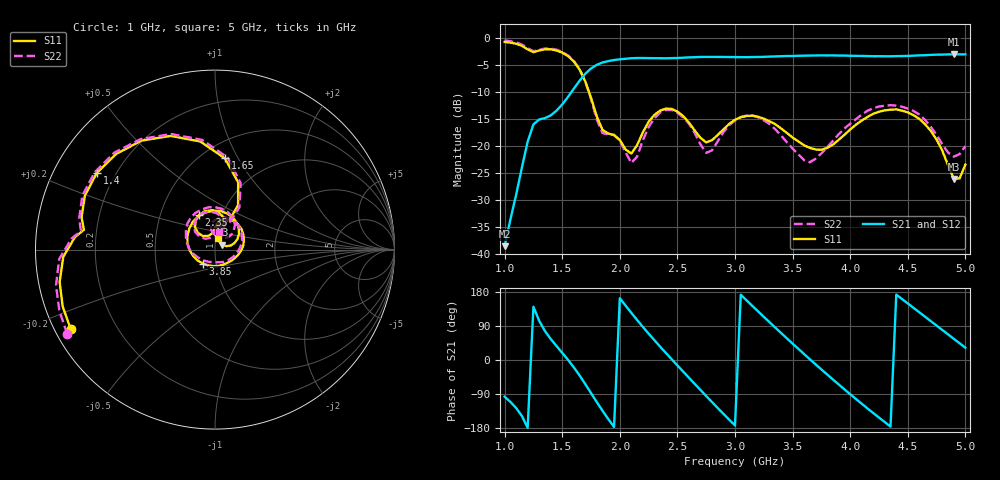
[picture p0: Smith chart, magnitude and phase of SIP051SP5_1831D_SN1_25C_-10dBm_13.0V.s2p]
# GHz  S  dB  R  50
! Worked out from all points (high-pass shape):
!   81 points, 1 GHz to 5 GHz, reference 50 ohm
!   highest |S21| = -3.03 dB at 4.9 GHz (marker M1); lowest = -38.6 dB at 1 GHz (marker M2)
!   |S21| within 3 dB of the highest: 1.731 GHz to end of sweep
!   lowest |S11| = -26.1 dB at 4.9 GHz (marker M3), VSWR 1.10, Z = 54.2 + j2.93 ohm
!   |S11| at or under -10 dB: 1.732 GHz to end of sweep
!   |S22| runs from -23.2 to -0.5 dB; largest |S21 - S12| = 0.002
!   S11 on the Smith chart (normalised r, x): 1 GHz: 0.05, -0.26; 1.4 GHz: 0.13, +0.29; 1.65 GHz: 0.64, +0.88; 2.35 GHz: 0.78, +0.32; 3.85 GHz: 0.86, -0.14; 5 GHz: 1.03, +0.13
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1  -0.74 -151.1  -38.57 -96.8  -38.32 -95.6  -0.46 -150.3
1.25  -2.63 171.4  -16.02 140.4  -16.02 140.4  -2.45 172.1
1.4  -2.10 147.0  -14.35 55.6  -14.36 55.5  -1.98 147.3
1.65  -5.83 83.8  -7.94 -40.5  -7.94 -40.4  -5.71 82.2
1.7  -8.03 71.0  -6.64 -63.4  -6.65 -63.4  -8.02 68.9
1.85  -17.03 75.2  -4.54 -134.0  -4.54 -133.9  -17.62 76.6
2  -18.90 91.2  -3.96 163.1  -3.95 163.3  -19.04 87.5
2.15  -19.87 131.7  -3.72 105.7  -3.72 105.7  -22.00 130.9
2.35  -13.46 114.6  -3.75 35.2  -3.76 35.3  -13.83 120.0
2.5  -13.63 85.0  -3.71 -14.3  -3.71 -14.3  -13.84 87.4
2.7  -18.50 70.4  -3.52 -79.0  -3.53 -79.0  -19.71 68.0
3  -15.16 74.5  -3.55 -172.6  -3.54 -172.6  -15.28 86.0
3.15  -14.40 47.5  -3.54 142.9  -3.54 142.9  -14.34 54.2
3.35  -15.99 7.9  -3.42 85.5  -3.43 85.5  -16.92 6.2
3.55  -19.17 -34.8  -3.30 29.5  -3.30 29.5  -21.55 -55.1
3.7  -20.66 -77.2  -3.25 -11.6  -3.25 -11.5  -22.36 -116.4
3.85  -19.77 -130.8  -3.23 -51.5  -3.23 -51.5  -19.07 -160.8
4.05  -16.07 167.0  -3.32 -102.9  -3.31 -102.8  -15.04 156.2
4.35  -13.29 93.4  -3.40 -175.7  -3.40 -175.7  -12.45 99.0
4.65  -15.98 32.7  -3.20 114.2  -3.18 114.3  -15.18 50.6
4.9  -26.11 33.0  -3.03 55.7  -3.03 55.8  -21.99 59.6
5  -23.46 73.4  -3.04 32.4  -3.04 32.6  -20.04 76.9
